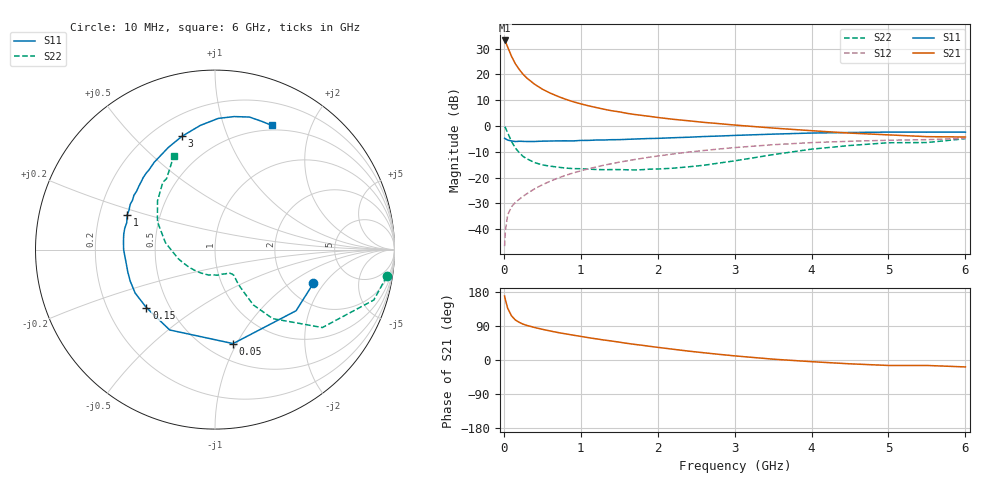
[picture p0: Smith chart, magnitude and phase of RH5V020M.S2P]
! SIEMENS Small Signal Semiconductors
! BFR106
! Si NPN RF Bipolar Junction Transistor in SOT23
! VCE = 5 V  IC = 20 mA
! Common Emitter S-Parameters:  August  1996
# GHz  S  MA  R  50
!  f  S11  S21  S12  S22
! GHz  MAG  ANG  MAG  ANG  MAG  ANG  MAG  ANG
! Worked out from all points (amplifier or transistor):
!   36 points, 10 MHz to 6 GHz, reference 50 ohm
!   highest |S21| = 33.2 dB at 10 MHz (marker M1)
!   |S21| within 3 dB of that: start of sweep to 55.95 MHz
!   unconditionally stable (mu >= 1): 370.3 MHz to 2.11 GHz
!   at 250 MHz: K = 0.89, MSG = 23.7 dB, |S12| = -27.2 dB
!   at 1.4 GHz: K = 1.07, MAG = 8.7 dB, |S12| = -14.6 dB
!   at 6 GHz: K = 0.99, MSG = 0.3 dB, |S12| = -4.8 dB
!   S11 on the Smith chart (normalised r, x): 10 MHz: 2.78, -1.57; 50 MHz: 0.66, -0.97; 150 MHz: 0.37, -0.32; 1 GHz: 0.32, +0.17; 3 GHz: 0.32, +0.70; 6 GHz: 0.45, +1.46
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0.01  0.5797 -18.8  45.49 168.6  0.0047 83.3  0.9683 -8.9
0.02  0.5659 -37.0  43.25 159.2  0.0093 76.5  0.9284 -17.6
0.05  0.5333 -79.1  33.82 136.4  0.019 61.7  0.7391 -36.0
0.1  0.514 -119.4  22.41 116.5  0.0273 54.4  0.5011 -50.1
0.15  0.5007 -139.8  16.05 105.6  0.0331 53.9  0.3746 -55.3
0.2  0.5065 -151.4  12.49 99.4  0.0381 56.8  0.3053 -55.7
0.25  0.504 -159.5  10.08 94.6  0.0435 58.4  0.2574 -56.0
0.3  0.5017 -165.2  8.484 91.2  0.0489 60.8  0.2316 -56.0
0.4  0.5017 -173.6  6.452 85.8  0.0607 63.7  0.1958 -54.7
0.5  0.5091 180.0  5.184 81.0  0.0727 65.3  0.1765 -53.8
0.6  0.5119 175.0  4.362 76.7  0.0849 66.2  0.1671 -54.9
0.7  0.5157 170.4  3.772 72.6  0.0977 66.7  0.16 -56.7
0.8  0.5166 166.7  3.313 69.1  0.1102 66.4  0.1532 -58.4
1  0.5261 158.3  2.688 62.3  0.1354 65.7  0.1488 -63.4
1.1  0.5269 155.5  2.465 58.9  0.1483 65.0  0.1464 -67.5
1.6  0.5519 140.3  1.761 44.0  0.2115 60.2  0.142 -88.6
2.2  0.5929 124.8  1.351 28.4  0.2875 52.8  0.1523 -121.0
3  0.6575 106.2  1.045 10.9  0.3819 41.2  0.2114 -166.3
3.5  0.6965 96.8  0.913 2.2  0.4347 33.6  0.2791 172.0
4.5  0.7488 81.8  0.729 -10.1  0.5065 17.8  0.4196 139.8
5.5  0.7606 69.5  0.622 -14.4  0.544 7.2  0.4786 124.3
6  0.7607 65.4  0.613 -18.3  0.5775 -0.4  0.5686 113.9
